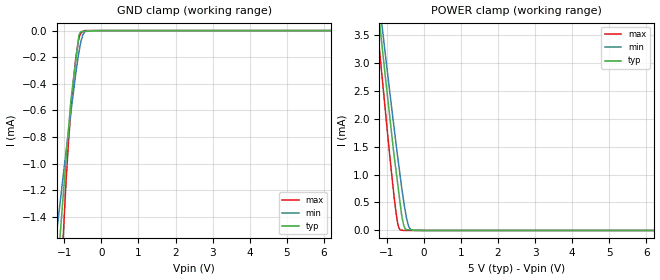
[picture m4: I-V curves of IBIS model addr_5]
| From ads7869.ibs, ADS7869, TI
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|   addr_5 Model
[Model]   addr_5
Model_type   Input
Vinl = 1.5
Vinh = 3.5
|   typ   min   max
|   (nom PVT)   (fast PVT)   (slow PVT)
|C_comp from frequency sweep method (F=8MHz)
|Average
|C_comp   2.263e-12   2.188e-12   2.339e-12
|C_comp from LC tank measurement(L=1nH)
|Average
|Resonant Frequency(Hz)   3.590e+09   3.640e+09   3.550e+09
C_comp   1.967e-12   1.914e-12   2.012e-12
| Where nom  PVT is Nominal Process, 5V, 36C
|   Fast PVT is Strong Process,  5.5V, -40C
|   Slow PVT is Weak Process,   4.5V, 96C
[Model Spec]
|Subparameter   typ   min   max
Vinh   3.5   3.15   3.85
Vinl   1.5   1.35   1.65
[Voltage Range]   5   4.5   5.5
|Ambient Temperature   25   85   -40
|Junction Temperature
[Temperature Range]   36   96   -40
[Power Clamp Reference]   5   4.5   5.5
[GND Clamp Reference]   0   0   0
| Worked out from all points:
|   GND clamp passes 1 mA (typ) near -0.96 V on its own axis
|   POWER clamp passes 1 mA (typ) near -0.74 V on its own axis
[GND Clamp]
|   Voltage   I(typ)   I(min)   I(max)
-5V       -16.41mA   -11.09mA   -29.33mA
-1.247V   -2.029mA   -1.615mA   -2.916mA
-1.123V   -1.575mA   -1.314mA   -2.112mA
-1.024V   -1.215mA   -1.076mA   -1.513mA
-957.5mV  -983.3uA   -920uA     -1.155mA
-891.5mV  -755.8uA   -765uA     -853.6uA
-792.5mV  -455.7uA   -546.9uA   -496.5uA
-693.5mV  -232.1uA   -328.9uA   -215.8uA
-605mV    -32.28uA   -159.9uA   -58.48uA
-545mV    -7.389uA   -74.83uA   -13.56uA
-392mV    -5.314uA   -1.095uA   0A
10V       0A         0A         0A
[POWER Clamp]
|   Voltage   I(typ)   I(min)   I(max)
-5V       28.13mA    26.55mA    30.5mA
-1.249V   4.043mA    4.343mA    3.579mA
-1.036V   2.721mA    3.123mA    2.114mA
-869.5mV  1.726mA    2.194mA    1.008mA
-748.5mV  1.054mA    1.537mA    303.7uA
-704.5mV  823uA      1.303mA    119.5uA
-638.5mV  476.2uA    966.3uA    8.772uA
-600mV    279.8uA    772.2uA    5.16uA
-540mV    88.21uA    499.5uA    0A
-414.5mV  13.96uA    82.68uA    0A
-239mV    8.048uA    0A         0A
10V       0A         0A         0A
